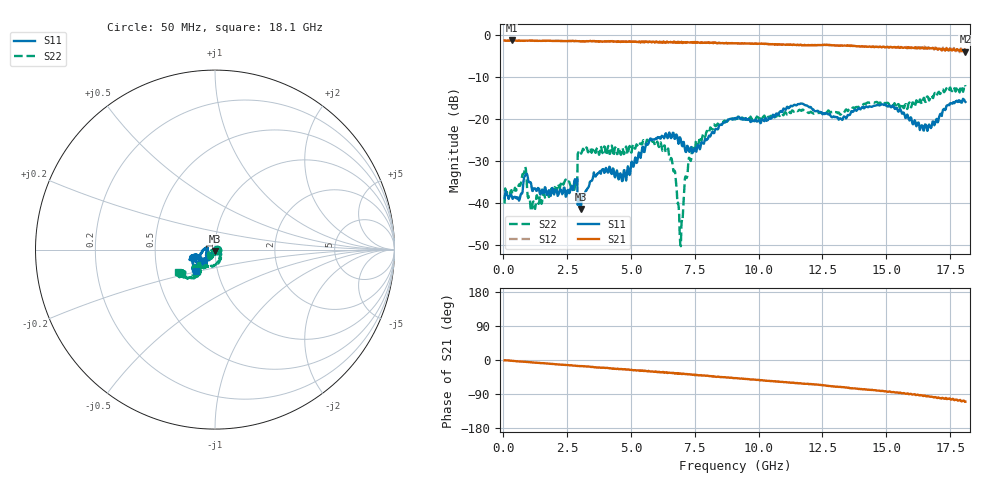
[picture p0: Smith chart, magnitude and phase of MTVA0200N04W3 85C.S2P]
! Network Analyzer HP8720D.06.14 Serial No. US36140669
! 17 Jan 2005  13:07:21
! Frequency  S11  S21  S12  S22
# HZ  S  DB R 50
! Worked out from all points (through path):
!   801 points, 50 MHz to 18.1 GHz, reference 50 ohm
!   highest |S21| = -1.36 dB at 320.8 MHz (marker M1); lowest = -4.0 dB at 18.1 GHz (marker M2)
!   group delay of S21, straight-line fit = 15.9 ps
!   lowest |S11| = -41.4 dB at 3.028 GHz (marker M3), VSWR 1.02, Z = 49.8 - j0.822 ohm
!   |S11| at or under -10 dB: start of sweep to end of sweep
!   |S22| runs from -50.2 to -11.9 dB; largest |S21 - S12| = 0.033
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5e7  -38.86 -23.7  -1.38 -0.8  -1.40 -1.0  -40.11 -10.4
3.2075e8  -38.10 -24.2  -1.36 -2.0  -1.36 -2.4  -36.93 -34.2
6.591875e8  -38.52 -9.9  -1.45 -3.8  -1.44 -4.3  -35.90 -50.2
8.17125e8  -33.83 -12.8  -1.44 -4.4  -1.42 -4.9  -32.73 -72.7
1.155562e9  -37.13 -49.9  -1.41 -6.5  -1.41 -6.9  -39.82 -95.0
2.351375e9  -36.92 -64.9  -1.52 -12.6  -1.50 -12.9  -35.63 -121.1
2.734938e9  -36.88 -67.3  -1.48 -14.8  -1.51 -15.2  -36.71 -139.8
3.02825e9  -41.41 -103.6  -1.59 -16.2  -1.58 -16.7  -28.10 -107.5
3.073375e9  -39.06 -95.9  -1.56 -16.3  -1.53 -16.5  -27.93 -105.2
3.614875e9  -33.70 -85.0  -1.56 -19.0  -1.55 -19.5  -28.07 -116.3
4.743e9  -32.18 -115.8  -1.69 -24.2  -1.66 -25.0  -28.24 -114.8
6.074188e9  -24.37 -128.1  -1.86 -32.2  -1.84 -32.4  -26.40 -135.3
6.63825e9  -23.30 -124.8  -1.84 -34.5  -1.81 -35.2  -31.33 -164.1
6.954125e9  -25.01 -152.3  -1.83 -35.6  -1.85 -35.8  -50.24 50.3
7.17975e9  -27.24 -160.4  -1.86 -36.7  -1.77 -37.6  -34.06 -30.6
7.473062e9  -27.22 173.6  -1.72 -38.9  -1.79 -39.6  -27.48 -48.6
9.075e9  -19.83 -148.3  -2.06 -47.7  -2.06 -48.2  -20.11 -111.4
1.209838e10  -17.64 -151.1  -2.44 -64.2  -2.46 -64.5  -18.52 -138.8
1.320394e10  -19.87 -150.1  -2.59 -71.0  -2.56 -71.6  -19.00 -134.4
1.509919e10  -16.96 -138.2  -3.05 -83.6  -2.98 -84.4  -16.45 -142.1
1.654319e10  -21.36 -136.2  -3.09 -94.7  -3.35 -96.2  -15.97 -125.1
1.81e10  -15.97 -131.9  -4.03 -110.1  -3.83 -111.4  -12.28 -148.7
